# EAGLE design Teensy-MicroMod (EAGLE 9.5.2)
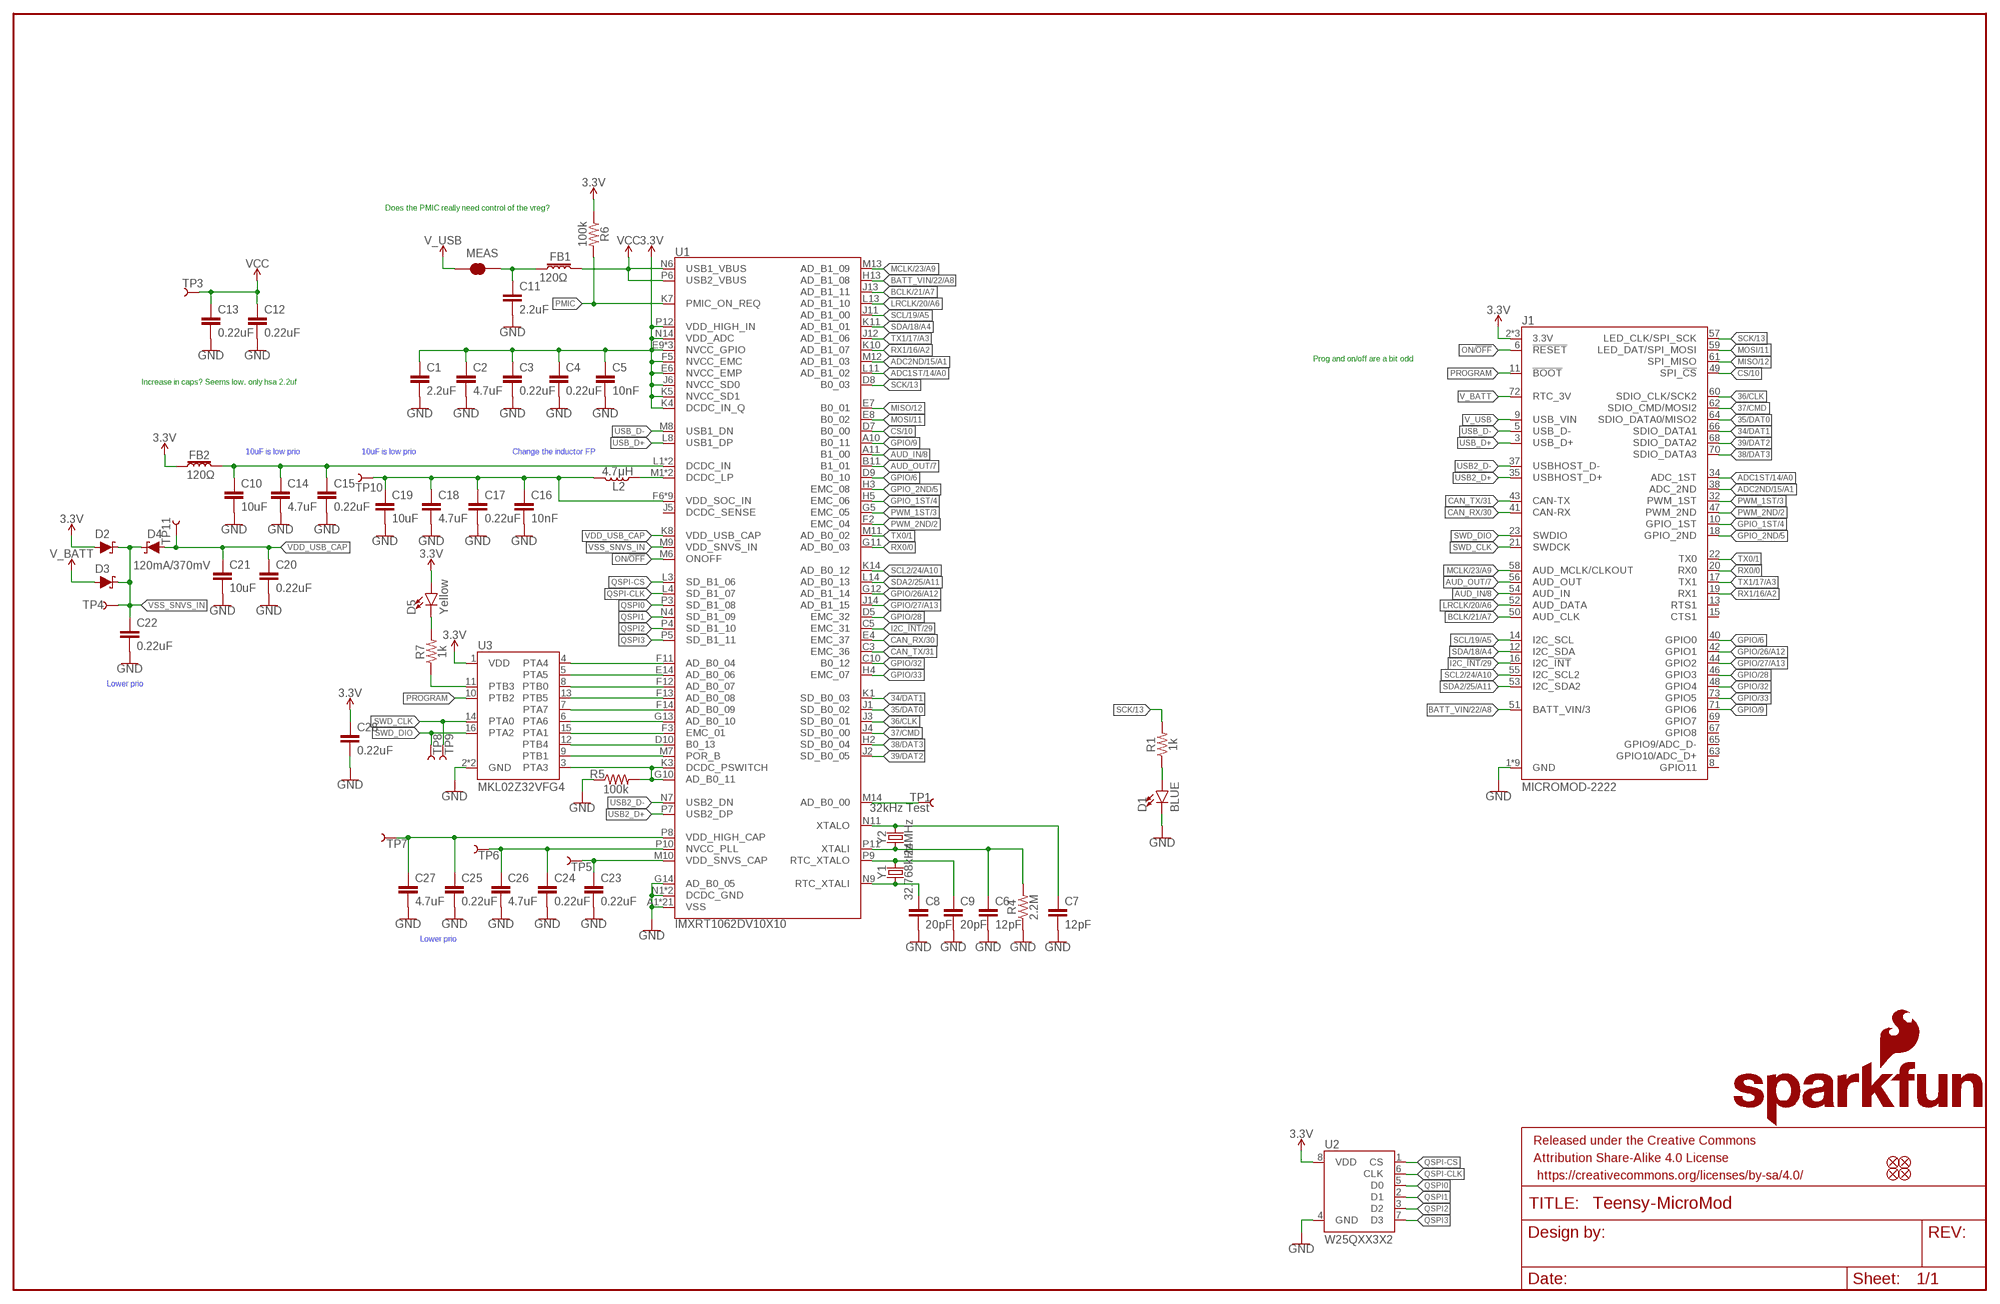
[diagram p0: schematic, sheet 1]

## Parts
C1  2.2uF  2.2UF-0402_TIGHT-10V-10%-X5R  [0402-TIGHT]
C2  4.7uF  4.7UF-0402_TIGHT-6.3V-20%-X5R  [0402-TIGHT]
C3  0.22uF  0.22UF-0402T-10V-10%  [0402-TIGHT]
C4  0.22uF  0.22UF-0402T-10V-10%  [0402-TIGHT]
C5  10nF  10NF-0402T-25V-10%  [0402-TIGHT]
C6  12pF  12PF-0402T-50V-5%  [0402-TIGHT]
C7  12pF  12PF-0402T-50V-5%  [0402-TIGHT]
C8  20pF  20PF-0402T-50V-5%  [0402-TIGHT]
C9  20pF  20PF-0402T-50V-5%  [0402-TIGHT]
C10  10uF  10UF-0402T-6.3V-20%  [0402-TIGHT]
C11  2.2uF  2.2UF-0402_TIGHT-10V-10%-X5R  [0402-TIGHT]
C12  0.22uF  0.22UF-0402T-10V-10%  [0402-TIGHT]
C13  0.22uF  0.22UF-0402T-10V-10%  [0402-TIGHT]
C14  4.7uF  4.7UF-0402_TIGHT-6.3V-20%-X5R  [0402-TIGHT]
C15  0.22uF  0.22UF-0402T-10V-10%  [0402-TIGHT]
C16  10nF  10NF-0402T-25V-10%  [0402-TIGHT]
C17  0.22uF  0.22UF-0402T-10V-10%  [0402-TIGHT]
C18  4.7uF  4.7UF-0402_TIGHT-6.3V-20%-X5R  [0402-TIGHT]
C19  10uF  10UF-0402T-6.3V-20%  [0402-TIGHT]
C20  0.22uF  0.22UF-0402T-10V-10%  [0402-TIGHT]
C21  10uF  10UF-0402T-6.3V-20%  [0402-TIGHT]
C22  0.22uF  0.22UF-0402T-10V-10%  [0402-TIGHT]
C23  0.22uF  0.22UF-0402T-10V-10%  [0402-TIGHT]
C24  0.22uF  0.22UF-0402T-10V-10%  [0402-TIGHT]
C25  0.22uF  0.22UF-0402T-10V-10%  [0402-TIGHT]
C26  4.7uF  4.7UF-0402_TIGHT-6.3V-20%-X5R  [0402-TIGHT]
C27  4.7uF  4.7UF-0402_TIGHT-6.3V-20%-X5R  [0402-TIGHT]
C28  0.22uF  0.22UF-0402T-10V-10%  [0402-TIGHT]
D1  BLUE  LED-BLUE0603  [LED-0603]
D2  120mA370mV  DIODE-SCHOTTKY-RB751S40  [SOD-523]
D3  120mA/370mV  DIODE-SCHOTTKY-RB751S40  [SOD-523]
D4  120mA/370mV  DIODE-SCHOTTKY-RB751S40  [SOD-523]
D5  Yellow  LED-YELLOW0603  [LED-0603]
FB1  120Ω  FERRITE_BEAD-120_OHM-0402  [0402]
FB2  120Ω  FERRITE_BEAD-120_OHM-0402  [0402]
FD1  FIDUCIALUFIDUCIAL  [FIDUCIAL-MICRO]
FD2  FIDUCIALUFIDUCIAL  [FIDUCIAL-MICRO]
FD3  FIDUCIALUFIDUCIAL  [FIDUCIAL-MICRO]
FD4  FIDUCIALUFIDUCIAL  [FIDUCIAL-MICRO]
FRAME1  FRAME-LEDGER  [CREATIVE_COMMONS]
J1  MICROMOD-2222  [M.2-CARD-E-22]
L2  4.7μH  4.7μH_SHIELDED_INDUCTOR  [1008(2520)]
LOGO1  SFE_LOGO_NAME_FLAME.1_INCH  [SFE_LOGO_NAME_FLAME_.1]
MEAS  JUMPER-SMT_2_NC_TRACE_SILK  [SMT-JUMPER_2_NC_TRACE_SILK]
R1  1k  1KOHM-0402T-1/16W-1%  [0402-TIGHT]
R4  2.2M  2.2MOHMS-0402T-1/10W-1%  [0402-TIGHT]
R5  100k  100KOHM-0402T-1/16W-1%  [0402-TIGHT]
R6  100k  100KOHM-0402T-1/16W-1%  [0402-TIGHT]
R7  1k  1KOHM-0402T-1/16W-1%  [0402-TIGHT]
TP1  32kHz Test  TEST-POINT2  [PAD.02X.02]
TP3  TEST-POINT2  [PAD.02X.02]
TP4  TEST-POINT2  [PAD.02X.02]
TP5  TEST-POINT2  [PAD.02X.02]
TP6  TEST-POINT2  [PAD.02X.02]
TP7  TEST-POINT2  [PAD.02X.02]
TP8  TEST-POINT2  [PAD.02X.02]
TP9  TEST-POINT2  [PAD.02X.02]
TP10  TEST-POINT2  [PAD.02X.02]
TP11  TEST-POINT2  [PAD.02X.02]
U1  IMXRT1062DV10X10  [IMXRT1062]
U2  W25QXX3X2  [USON-8]
U3  MKL02Z32VFG4  MKL02Z32VFG4QFN-16  [QFN-16]
Y1  32.768kHz  CRYSTAL-32.768KHZSMD-3.2X1.5  [CRYSTAL-SMD-3.2X1.5MM]
Y2  24MHz  CRYSTAL-24MHZ-SMD-2.0X1.6MM  [CRYSTAL-SMD-2.0X1.6MM]

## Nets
3.3V: C1.1 C2.1 C3.1 C4.1 C5.1 C28.1 D2.A D5.A FB2.1 J1.2(3.3V) J1.4(3.3V) J1.74(3.3V) R6.1 U1.E6(NVCC_EMP) U1.E9(NVCC_GPIO) U1.F5(NVCC_EMC) U1.F10(NVCC_GPIO) U1.J6(NVCC_SD0) U1.J10(NVCC_GPIO) U1.K4(DCDC_IN_Q) U1.K5(NVCC_SD1) U1.N14(VDD_ADC) U1.P12(VDD_HIGH_IN) U2.8(VDD) U3.1(VDD)
34/DAT1: J1.66(SDIO_DATA1) U1.K1(SD_B0_03)
35/DAT0: J1.64(SDIO_DATA0/MISO2) U1.J1(SD_B0_02)
36/CLK: J1.60(SDIO_CLK/SCK2) U1.J3(SD_B0_01)
37/CMD: J1.62(SDIO_CMD/MOSI2) U1.J4(SD_B0_00)
38/DAT3: J1.70(SDIO_DATA3) U1.H2(SD_B0_04)
39/DAT2: J1.68(SDIO_DATA2) U1.J2(SD_B0_05)
ADC1ST/14/A0: J1.34(ADC_1ST) U1.L11(AD_B1_02)
ADC2ND/15/A1: J1.38(ADC_2ND) U1.M12(AD_B1_03)
AUD_IN/8: J1.54(AUD_IN) U1.A11(B1_00)
AUD_OUT/7: J1.56(AUD_OUT) U1.B11(B1_01)
BATT_VIN/22/A8: J1.51(BATT_VIN/3) U1.H13(AD_B1_08)
BCLK/21/A7: J1.50(AUD_CLK) U1.J13(AD_B1_11)
BOOTMODE0: U1.F11(AD_B0_04) U3.4(PTA4)
CAN_RX/30: J1.41(CAN-RX) U1.E4(EMC_37)
CAN_TX/31: J1.43(CAN-TX) U1.C3(EMC_36)
CS/10: J1.49(SPI_!CS!) U1.D7(B0_00)
DEBUG_EN: U1.F3(EMC_01) U3.15(PTA1)
DEBUG_SWO: U1.D10(B0_13) U3.12(PTB4)
GND: C1.2 C2.2 C3.2 C4.2 C5.2 C6.2 C7.2 C8.2 C9.2 C10.2 C11.2 C12.2 C13.2 C14.2 C15.2 C16.2 C17.2 C18.2 C19.2 C20.2 C21.2 C22.2 C23.2 C24.2 C25.2 C26.2 C27.2 C28.2 D1.C J1.1(GND) J1.7(GND) J1.33(GND) J1.36(GND) J1.39(GND) J1.45(GND) J1.75(GND) J1.GND J1.GND-SM-B(GND) R4.1 R5.1 U1.A1(VSS) U1.A14(VSS) U1.B5(VSS) U1.B10(VSS) U1.E2(VSS) U1.E13(VSS) U1.G7(VSS) U1.G8(VSS) U1.G14(AD_B0_05) U1.H7(VSS) U1.H8(VSS) U1.J7(VSS) U1.J8(VSS) U1.K2(VSS) U1.K6(VSS) U1.K9(VSS) U1.K13(VSS) U1.L9(VSS) U1.N1(DCDC_GND) U1.N2(DCDC_GND) U1.N5(VSS) U1.N8(VSS) U1.P1(VSS) U1.P14(VSS) U2.4(GND) U3.2(GND) U3.17(GND)
GPIO/6: J1.40(GPIO0) U1.D9(B0_10)
GPIO/9: J1.71(GPIO6) U1.A10(B0_11)
GPIO/26/A12: J1.42(GPIO1) U1.G12(AD_B1_14)
GPIO/27/A13: J1.44(GPIO2) U1.J14(AD_B1_15)
GPIO/28: J1.46(GPIO3) U1.D5(EMC_32)
GPIO/32: J1.48(GPIO4) U1.C10(B0_12)
GPIO/33: J1.73(GPIO5) U1.H4(EMC_07)
GPIO_1ST/4: J1.10(GPIO_1ST) U1.H5(EMC_06)
GPIO_2ND/5: J1.18(GPIO_2ND) U1.H3(EMC_08)
I2C_!INT!/29: J1.16(I2C_!INT!) U1.C5(EMC_31)
JTAG_MOD: U1.F13(AD_B0_08) U3.13(PTB5)
JTAG_TCK: U1.F12(AD_B0_07) U3.8(PTB0)
JTAG_TDI: U1.F14(AD_B0_09) U3.7(PTA7)
JTAG_TDO: U1.G13(AD_B0_10) U3.6(PTA6)
JTAG_TMS: U1.E14(AD_B0_06) U3.5(PTA5)
JTAG_TRST: R5.2 U1.G10(AD_B0_11) U1.K3(DCDC_PSWITCH) U3.3(PTA3)
LRCLK/20/A6: J1.52(AUD_DATA) U1.L13(AD_B1_10)
MCLK/23/A9: J1.58(AUD_MCLK/CLKOUT) U1.M13(AD_B1_09)
MISO/12: J1.61(SPI_MISO) U1.E7(B0_01)
MOSI/11: J1.59(LED_DAT/SPI_MOSI) U1.E8(B0_02)
N$1: TP1.P$1 U1.M14(AD_B0_00)
N$2: D1.A R1.1
N$3: C10.1 C14.1 C15.1 FB2.2 U1.L1(DCDC_IN) U1.L2(DCDC_IN)
N$4: C7.1 U1.N11(XTALO) Y2.3
N$5: C6.1 R4.2 U1.P11(XTALI) Y2.1
N$9: L2.1 U1.M1(DCDC_LP) U1.M2(DCDC_LP)
N$10: C11.1 FB1.1 MEAS.2
N$12: R7.1 U3.11(PTB3)
N$13: D5.C R7.2
N$30: C23.1 TP5.P$1 U1.M10(VDD_SNVS_CAP)
N$31: C9.1 U1.P9(RTC_XTALO) Y1.P$2
N$32: C8.1 U1.N9(RTC_XTALI) Y1.P$1
N$33: C24.1 C26.1 TP6.P$1 U1.P10(NVCC_PLL)
N$34: C25.1 C27.1 TP7.P$1 U1.P8(VDD_HIGH_CAP)
ON/!OFF!: J1.6(!RESET!) U1.M6(ONOFF)
PMIC: R6.2 U1.K7(PMIC_ON_REQ)
PORB_RESET: U1.M7(POR_B) U3.9(PTB1)
PROGRAM: J1.11(!BOOT!) U3.10(PTB2)
PWM_1ST/3: J1.32(PWM_1ST) U1.G5(EMC_05)
PWM_2ND/2: J1.47(PWM_2ND) U1.F2(EMC_04)
QSPI0: U1.P3(SD_B1_08) U2.5(D0)
QSPI1: U1.N4(SD_B1_09) U2.2(D1)
QSPI2: U1.P4(SD_B1_10) U2.3(D2)
QSPI3: U1.P5(SD_B1_11) U2.7(D3)
QSPI-CLK: U1.L4(SD_B1_07) U2.6(CLK)
QSPI-CS: U1.L3(SD_B1_06) U2.1(CS)
RX0/0: J1.20(RX0) U1.G11(AD_B0_03)
RX1/16/A2: J1.19(RX1) U1.K10(AD_B1_07)
SCK/13: J1.57(LED_CLK/SPI_SCK) R1.2 U1.D8(B0_03)
SCL2/24/A10: J1.55(I2C_SCL2) U1.K14(AD_B0_12)
SCL/19/A5: J1.14(I2C_SCL) U1.J11(AD_B1_00)
SDA2/25/A11: J1.53(I2C_SDA2) U1.L14(AD_B0_13)
SDA/18/A4: J1.12(I2C_SDA) U1.K11(AD_B1_01)
SWD_CLK: J1.21(SWDCK) TP9.P$1 U3.14(PTA0)
SWD_DIO: J1.23(SWDIO) TP8.P$1 U3.16(PTA2)
TX0/1: J1.22(TX0) U1.M11(AD_B0_02)
TX1/17/A3: J1.17(TX1) U1.J12(AD_B1_06)
USB2_D+: J1.35(USBHOST_D+) U1.P7(USB2_DP)
USB2_D-: J1.37(USBHOST_D-) U1.N7(USB2_DN)
USB_D+: J1.3(USB_D+) U1.L8(USB1_DP)
USB_D-: J1.5(USB_D-) U1.M8(USB1_DN)
V_BATT: D3.A J1.72(RTC_3V)
V_USB: J1.9(USB_VIN) MEAS.1
VCC: C12.1 C13.1 FB1.2 TP3.P$1 U1.N6(USB1_VBUS) U1.P6(USB2_VBUS)
VDD_SOC_IN: C16.1 C17.1 C18.1 C19.1 L2.2 TP10.P$1 U1.F6(VDD_SOC_IN) U1.F7(VDD_SOC_IN) U1.F8(VDD_SOC_IN) U1.F9(VDD_SOC_IN) U1.G6(VDD_SOC_IN) U1.G9(VDD_SOC_IN) U1.H6(VDD_SOC_IN) U1.H9(VDD_SOC_IN) U1.J9(VDD_SOC_IN)
VDD_USB_CAP: C20.1 C21.1 D4.A TP11.P$1 U1.K8(VDD_USB_CAP)
VSS_SNVS_IN: C22.1 D2.C D3.C D4.C TP4.P$1 U1.M9(VDD_SNVS_IN)
Unconnected: J1.8(GPIO11) J1.13(RTS1) J1.15(CTS1) J1.63(GPIO10/ADC_D+) J1.65(GPIO9/ADC_D-) J1.67(GPIO8) J1.69(GPIO7) U1.J5(DCDC_SENSE)

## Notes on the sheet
- Does the PMIC really need control of the vreg?
- Prog and on/off are a bit odd
- Increase in caps? Seems low. only hsa 2.2uf
- 10uF is low prio | 10uF is low prio | Change the inductor FP
- Lower prio
- Lower prio

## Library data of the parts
C1 C11 = SparkFun-Capacitors:2.2UF: 2.2µF ceramic capacitors; PROD_ID: CAP-14232
C2 C14 C18 C26 C27 = SparkFun-Capacitors:4.7UF: 4.7µF ceramic capacitors; PROD_ID: CAP-14240
C3 C4 C12 C13 C15 C17 C20 C22-C25 C28 = SparkFun-Capacitors:0.22UF: 0.22µF ceramic capacitors; PROD_ID: CAP-14846
C5 C16 = SparkFun-Capacitors:10NF: 0.01uF/10nF/10,000pF ceramic capacitors; PROD_ID: CAP-14847
C6 C7 = SparkFun-Capacitors:12PF: 12pF ceramic capacitors; PROD_ID: CAP-14665
C8 C9 = SparkFun-Capacitors:20PF: 20pF ceramic capacitors; PROD_ID: CAP-14843
C10 C19 C21 = SparkFun-Capacitors:10UF: 10.0µF ceramic capacitors; PROD_ID: CAP-14848
D1 = SparkFun-LED:LED-BLUE: Blue SMD LED; PROD_ID: DIO-08575
D2-D4 = SparkFun-DiscreteSemi:DIODE-SCHOTTKY: Schottky diode; PROD_ID: DIO-11018; VALUE: 120mA/40V/370mV
D5 = SparkFun-LED:LED-YELLOW: Yellow SMD LED; PROD_ID: DIO-09003
FB1 FB2 = SparkFun-Coils:FERRITE_BEAD-120_OHM: Ferrite Bead (blocks, cores, rings, chokes, etc.); MFG_PART: BLM15HB121SN1D; PROD_ID: NDUC-14206
FD1-FD4 = SparkFun-Aesthetics:FIDUCIAL: Fiducial Alignment Points
FRAME1 = SparkFun-Aesthetics:FRAME-LEDGER: Schematic Frame - Ledger
J1 = Teensy:MICROMOD
L2 = SparkFun-Coils:4.7μH_SHIELDED_INDUCTOR: 4.7uH Inductor; PROD_ID: NDUC-14880
LOGO1 = SparkFun-Aesthetics:SFE_LOGO_NAME_FLAME: SparkFun Font Logo w/ Flame
MEAS = SparkFun-Jumpers:JUMPER-SMT_2_NC_TRACE: Normally closed trace jumper
R1 R7 = SparkFun-Resistors:1KOHM: 1kΩ resistor; PROD_ID: RES-14342
R4 = SparkFun-Resistors:2.2MOHMS: 2MΩ resistor; PROD_ID: RES-14844
R5 R6 = SparkFun-Resistors:100KOHM: 100kΩ resistor; PROD_ID: RES-13495
TP1 TP3-TP11 = SparkFun-Connectors:TEST-POINT: SparkFun Test Points
U1 = Teensy:IMXRT1062DV; PROD_ID: IC-14904
U2 = Teensy:W25QXX; PROD_ID: IC-14905
U3 = Teensy:MKL02Z32VFG4; PROD_ID: IC-14906
Y1 = SparkFun-Clocks:CRYSTAL-32.768KHZ: 32.768kHz Crystal; PROD_ID: XTAL-13062
Y2 = SparkFun-Clocks:CRYSTAL-24MHZ: 24MHz Crystal; PROD_ID: XTAL-14845

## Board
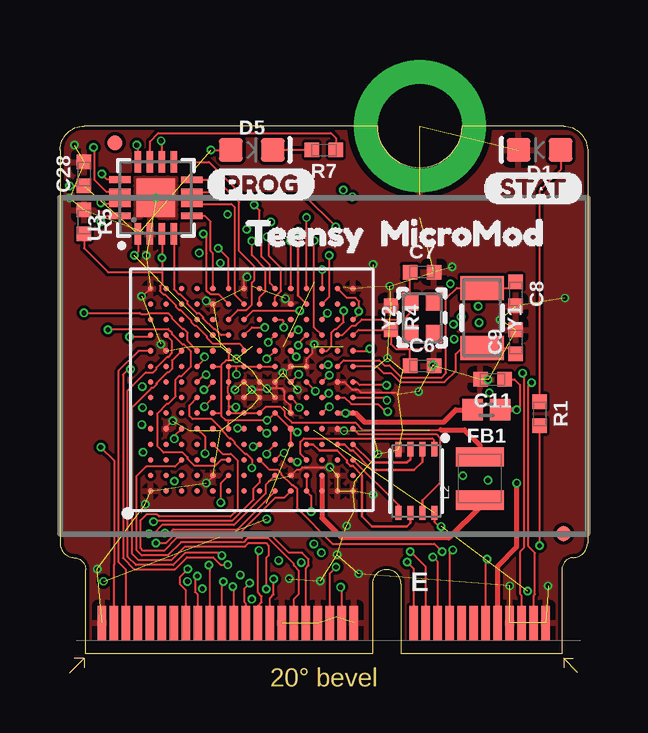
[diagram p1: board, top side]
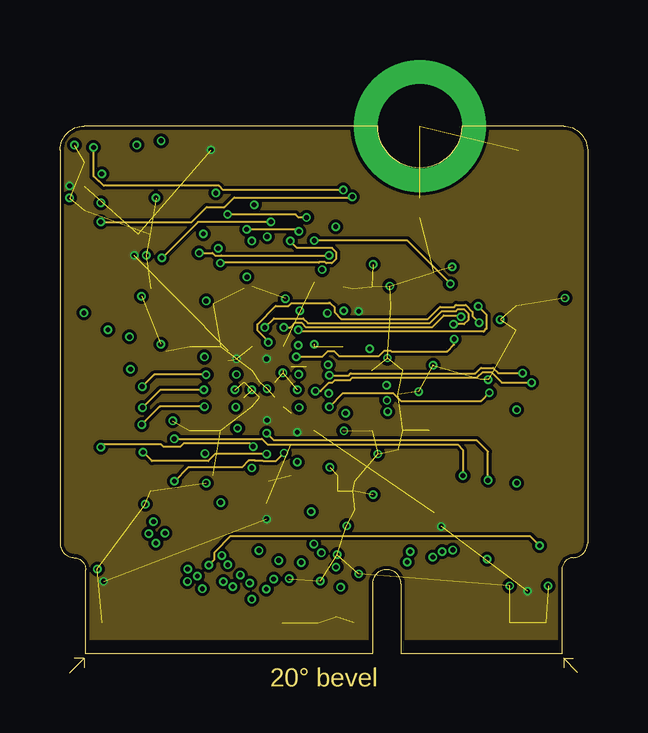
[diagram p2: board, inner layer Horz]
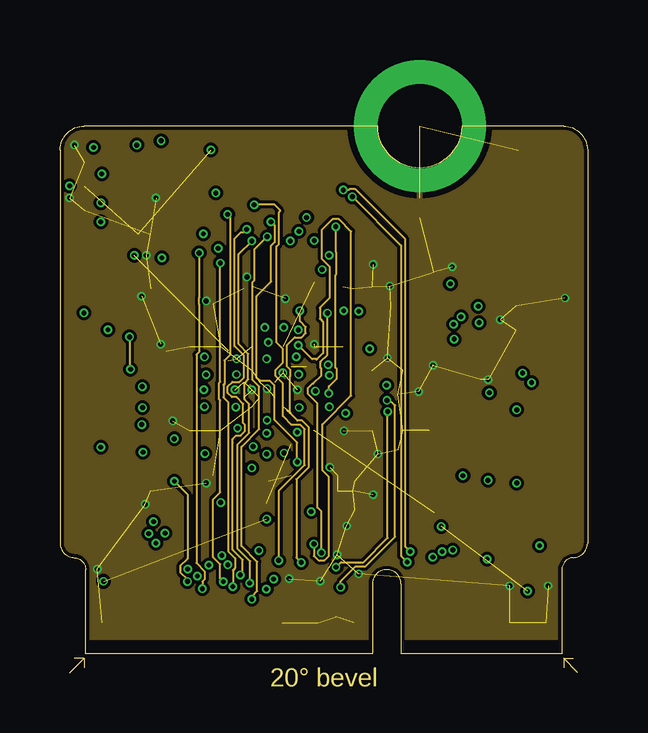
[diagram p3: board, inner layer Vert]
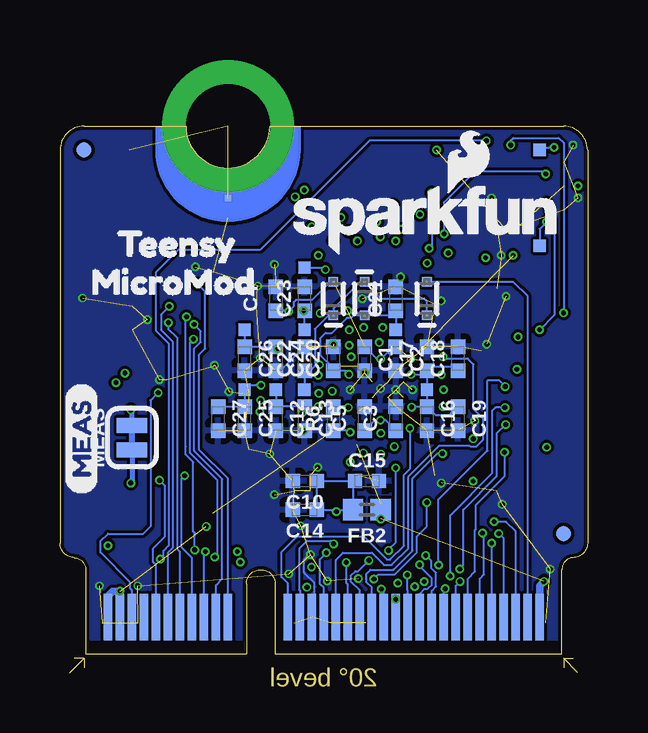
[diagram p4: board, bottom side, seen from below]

Size 22 x 22.8 mm. Coordinates in mm from the lower left corner, seen from the top.
Outline: 21.6,0 21,0.6
Outline: 21,0.6 21,0.2
Outline: 21,0.6 21.4,0.6
Outline: 0.4,0 1,0.6
Outline: 1,0.6 0.6,0.6
Outline: 1,0.6 1,0.2
Outline: 16.75,22.8 21,22.8 arc-87 22,21.8 22,5.4 arc-87 21.4,4.8 arc85 20.93,4.3 20.93,0.8 14.22,0.8 14.22,3.7 arc180 13.03,3.7 13.03,0.8 1.07,0.8 1.07,4.3 arc84 0.6,4.8 arc-87 0,5.4 0,21.8 arc-87 1,22.8 13.25,22.8
Outline: 16.75,22.8 arc-180 13.25,22.8
Outline: 16.75,22.8 arc-180 13.25,22.8
Copper layers (1+2*15+16): Top 0.035mm / dielectric 0.213359375mm / Horz 0.035mm / dielectric 1.0161mm / Vert 0.035mm / dielectric 0.213359375mm / Bottom 0.035mm
Design rules "SparkFun-4-layer-BGA-Extreme *": minimum track width 3.5mil, minimum drill 0.2mm, track to track 3.5mil, track to pad 3.5mil, pad to pad 3.5mil, via to via 3.5mil, smd to smd 0mil, copper to edge 4mil, drill to drill 4mil, minimum pad ring 3mil, minimum via ring 3mil, stop-mask expansion 4mil, vias tented up to drill 25mil, thermal gap 10mil

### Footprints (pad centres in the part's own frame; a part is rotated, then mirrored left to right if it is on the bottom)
0402-TIGHT = smd 0.6 x 0.6: 1 -0.5,0; 2 0.5,0
LED-0603 = smd 1 x 1: A -0.877,0; C 0.877,0
SOD-523 = smd 0.4 x 0.4: A -0.7,0; C 0.7,0
0402 = smd 0.85 x 0.9: 1 -0.58,0; 2 0.58,0
FIDUCIAL-MICRO = smd 0.635 x 0.635: 1 0,0
M.2-CARD-E-22 = smd 0.35 x 1.45: 1 9.25,1.275; 3 8.75,1.275; 5 8.25,1.275; 7 7.75,1.275; 9 7.25,1.275; 11 6.75,1.275; 13 6.25,1.275; 15 5.75,1.275; 17 5.25,1.275; 19 4.75,1.275; 21 4.25,1.275; 23 3.75,1.275; 33 1.25,1.275; 35 0.75,1.275; 37 0.25,1.275; 39 -0.25,1.275; 41 -0.75,1.275; 43 -1.25,1.275; 45 -1.75,1.275; 47 -2.25,1.275; 49 -2.75,1.275; 51 -3.25,1.275; 53 -3.75,1.275; 55 -4.25,1.275; 57 -4.75,1.275; 59 -5.25,1.275; 61 -5.75,1.275; 63 -6.25,1.275; 65 -6.75,1.275; 67 -7.25,1.275; 69 -7.75,1.275; 71 -8.25,1.275; 73 -8.75,1.275; 75 -9.25,1.275 | smd 0.35 x 1.95 bottom: 2 9,1.525; 4 8.5,1.525; 6 8,1.525; 8 7.5,1.525; 10 7,1.525; 12 6.5,1.525; 14 6,1.525; 16 5.5,1.525; 18 5,1.525; 20 4.5,1.525; 22 4,1.525; 32 1.5,1.525; 34 1,1.525; 36 0.5,1.525; 38 0,1.525; 40 -0.5,1.525; 42 -1,1.525; 44 -1.5,1.525; 46 -2,1.525; 48 -2.5,1.525; 50 -3,1.525; 52 -3.5,1.525; 54 -4,1.525; 56 -4.5,1.525; 58 -5,1.525; 60 -5.5,1.525; 62 -6,1.525; 64 -6.5,1.525; 66 -7,1.525; 68 -7.5,1.525; 70 -8,1.525; 72 -8.5,1.525; 74 -9,1.525 | drill 3.5 pad 5.5: GND 4,22 | smd 0.25 x 0.25 bottom: GND-SM-B 4,19
1008(2520) = smd 0.8 x 2: 1 -0.9,0; 2 0.9,0
SMT-JUMPER_2_NC_TRACE_SILK = smd 0.635 x 1.27: 1 -0.508,0; 2 0.508,0
PAD.02X.02 = smd 0.508 x 0.508: P$1 0,0
IMXRT1062 = smd 0.234 x 0.234: A1 -4.225,4.225; A2 -3.575,4.225; A3 -2.925,4.225; A4 -2.275,4.225; A5 -1.625,4.225; A6 -0.975,4.225; A7 -0.325,4.225; A8 0.325,4.225; A9 0.975,4.225; A10 1.625,4.225; A11 2.275,4.225; A12 2.925,4.225; A13 3.575,4.225; A14 4.225,4.225; B1 -4.225,3.575; B2 -3.575,3.575; B3 -2.925,3.575; B4 -2.275,3.575; B5 -1.625,3.575; B6 -0.975,3.575; B7 -0.325,3.575; B8 0.325,3.575; B9 0.975,3.575; B10 1.625,3.575; B11 2.275,3.575; B12 2.925,3.575; B13 3.575,3.575; B14 4.225,3.575; C1 -4.225,2.925; C2 -3.575,2.925; C3 -2.925,2.925; C4 -2.275,2.925; C5 -1.625,2.925; C6 -0.975,2.925; C7 -0.325,2.925; C8 0.325,2.925; C9 0.975,2.925; C10 1.625,2.925; C11 2.275,2.925; C12 2.925,2.925; C13 3.575,2.925; C14 4.225,2.925; D1 -4.225,2.275; D2 -3.575,2.275; D3 -2.925,2.275; D4 -2.275,2.275; D5 -1.625,2.275; D6 -0.975,2.275; D7 -0.325,2.275; D8 0.325,2.275; D9 0.975,2.275; D10 1.625,2.275; D11 2.275,2.275; D12 2.925,2.275; D13 3.575,2.275; D14 4.225,2.275; E1 -4.225,1.625; E2 -3.575,1.625; E3 -2.925,1.625; E4 -2.275,1.625; E5 -1.625,1.625; E6 -0.975,1.625; E7 -0.325,1.625; E8 0.325,1.625; E9 0.975,1.625; E10 1.625,1.625; E11 2.275,1.625; E12 2.925,1.625; E13 3.575,1.625; E14 4.225,1.625; F1 -4.225,0.975; F2 -3.575,0.975; F3 -2.925,0.975; F4 -2.275,0.975; F5 -1.625,0.975; F6 -0.975,0.975; F7 -0.325,0.975; F8 0.325,0.975; F9 0.975,0.975; F10 1.625,0.975; F11 2.275,0.975; F12 2.925,0.975; F13 3.575,0.975; F14 4.225,0.975; G1 -4.225,0.325; G2 -3.575,0.325; G3 -2.925,0.325; G4 -2.275,0.325; G5 -1.625,0.325; G6 -0.975,0.325; G7 -0.325,0.325; G8 0.325,0.325; G9 0.975,0.325; G10 1.625,0.325; G11 2.275,0.325; G12 2.925,0.325; G13 3.575,0.325; G14 4.225,0.325; H1 -4.225,-0.325; H2 -3.575,-0.325; H3 -2.925,-0.325; H4 -2.275,-0.325; H5 -1.625,-0.325; H6 -0.975,-0.325; H7 -0.325,-0.325; H8 0.325,-0.325; H9 0.975,-0.325; H10 1.625,-0.325; H11 2.275,-0.325; H12 2.925,-0.325; H13 3.575,-0.325; H14 4.225,-0.325; J1 -4.225,-0.975; J2 -3.575,-0.975; J3 -2.925,-0.975; J4 -2.275,-0.975; J5 -1.625,-0.975; J6 -0.975,-0.975; J7 -0.325,-0.975; J8 0.325,-0.975; J9 0.975,-0.975; J10 1.625,-0.975; J11 2.275,-0.975; J12 2.925,-0.975; J13 3.575,-0.975; J14 4.225,-0.975; K1 -4.225,-1.625; K2 -3.575,-1.625; K3 -2.925,-1.625; K4 -2.275,-1.625; K5 -1.625,-1.625; K6 -0.975,-1.625; K7 -0.325,-1.625; K8 0.325,-1.625; K9 0.975,-1.625; K10 1.625,-1.625; K11 2.275,-1.625; K12 2.925,-1.625; K13 3.575,-1.625; K14 4.225,-1.625; L1 -4.225,-2.275; L2 -3.575,-2.275; L3 -2.925,-2.275; L4 -2.275,-2.275; L5 -1.625,-2.275; L6 -0.975,-2.275; L7 -0.325,-2.275; L8 0.325,-2.275; L9 0.975,-2.275; L10 1.625,-2.275; L11 2.275,-2.275; L12 2.925,-2.275; L13 3.575,-2.275; L14 4.225,-2.275; M1 -4.225,-2.925; M2 -3.575,-2.925; M3 -2.925,-2.925; M4 -2.275,-2.925; M5 -1.625,-2.925; M6 -0.975,-2.925; M7 -0.325,-2.925; M8 0.325,-2.925; M9 0.975,-2.925; M10 1.625,-2.925; M11 2.275,-2.925; M12 2.925,-2.925; M13 3.575,-2.925; M14 4.225,-2.925; N1 -4.225,-3.575; N2 -3.575,-3.575; N3 -2.925,-3.575; N4 -2.275,-3.575; N5 -1.625,-3.575; N6 -0.975,-3.575; N7 -0.325,-3.575; N8 0.325,-3.575; N9 0.975,-3.575; N10 1.625,-3.575; N11 2.275,-3.575; N12 2.925,-3.575; N13 3.575,-3.575; N14 4.225,-3.575; P1 -4.225,-4.225; P2 -3.575,-4.225; P3 -2.925,-4.225; P4 -2.275,-4.225; P5 -1.625,-4.225; P6 -0.975,-4.225; P7 -0.325,-4.225; P8 0.325,-4.225; P9 0.975,-4.225; P10 1.625,-4.225; P11 2.275,-4.225; P12 2.925,-4.225; P13 3.575,-4.225; P14 4.225,-4.225
USON-8 = smd 0.6 x 0.25: 1 -1.325,0.75; 2 -1.325,0.25; 3 -1.325,-0.25; 4 -1.325,-0.75; 5 1.325,-0.75; 6 1.325,-0.25; 7 1.325,0.25; 8 1.325,0.75
QFN-16 = smd 0.9 x 0.29: 1 -1.5,0.75; 2 -1.5,0.25; 3 -1.5,-0.25; 4 -1.5,-0.75; 9 1.5,-0.75; 10 1.5,-0.25; 11 1.5,0.25; 12 1.5,0.75 | smd 0.29 x 0.9: 5 -0.75,-1.5; 6 -0.25,-1.5; 7 0.25,-1.5; 8 0.75,-1.5; 13 0.765,1.5; 14 0.25,1.5; 15 -0.25,1.5; 16 -0.75,1.5 | smd 1.6 x 1.6: 17 0,0
CRYSTAL-SMD-3.2X1.5MM = smd 1 x 1.8: P$1 -1.25,0; P$2 1.25,0
CRYSTAL-SMD-2.0X1.6MM = smd 0.75 x 0.7: 1 -0.675,-0.5; 2 0.675,-0.5; 3 0.675,0.5; 4 -0.675,0.5

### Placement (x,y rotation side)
C1  9.3,13.1 270 bottom
C2  8,13.1 270 bottom
C3  8,10.6 90 bottom
C4  13,15.6 90 bottom
C5  9.3,10.6 90 bottom
C6  15.1,12.8 0 top
C7  15.1,16.7 0 top
C8  19,15.8 270 top
C9  19,13.8 90 top
C10  11.8,8 180 bottom
C11  18.03,12.23 180 top
C12  13,10.6 270 bottom
C13  11.8,10.6 270 bottom
C14  11.8,6.8 180 bottom
C15  9.2,8 0 bottom
C16  6.7,10.6 270 bottom
C17  6.7,13.1 90 bottom
C18  5.4,13.1 90 bottom
C19  5.4,10.6 270 bottom
C20  10.6,13.1 90 bottom
C21  8,15.6 90 bottom
C22  11.8,13.1 90 bottom
C23  11.8,15.6 90 bottom
C24  13,13.1 270 bottom
C25  14.3,10.6 270 bottom
C26  14.3,13.1 270 bottom
C27  15.4,10.6 270 bottom
C28  1,20.8 90 top
D1  20,21.8 180 top
D2  10.6,15.6 270 bottom
D3  6.7,15.6 270 bottom
D4  9.3,15.6 90 bottom
D5  8,21.8 0 top
FB1  17.78,10.96 180 top
FB2  9.2,6.8 180 bottom
FD1  21,5.8 0 top
FD2  2.3,22.1 0 top
FD3  1,5.8 0 bottom
FD4  21,21.8 0 bottom
FRAME1  not placed on the board
J1  11,0.8 0 top
L2  17.5,8.1 90 top
LOGO1  6.7,18.9 0 bottom
MEAS  19,9.8 90 bottom
R1  20,10.8 270 top
R4  13.8,14.8 270 top
R5  1,18.8 270 top
R6  10.6,10.6 90 bottom
R7  11,21.8 180 top
TP1  11.8,16.9 270 bottom
TP3  13,11.8 90 bottom
TP4  11.81,11.8 0 bottom
TP5  11.8,14.3 0 bottom
TP6  14.3,14.3 0 bottom
TP7  14.3,11.8 0 bottom
TP8  2,17.8 0 bottom
TP9  2,21.8 0 bottom
TP10  6.7,11.8 270 bottom
TP11  8,14.3 270 bottom
U1  8,11.8 90 top
U2  14.86,7.99 270 top
U3  4,19.8 90 top
U$1  [TEENSY2]  20.5,17.9 0 bottom
U$2  [MICROMOD0]  12.45,18.33 0 top
U$3  [TEENSY2]  6.86,18.33 0 top
U$4  [PROG_32]  6.1,20.36 0 top
U$5  [MICROMOD0]  21.6,16.3 0 bottom
U$6  [STAT_32]  17.6,20.2 0 top
U$7  [MEAS_32]  21.1,7.4 90 bottom
Y1  17.6,14.8 270 top
Y2  15.1,14.8 90 top

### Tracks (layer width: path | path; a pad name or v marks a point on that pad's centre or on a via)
3.3V  (via drill 0.2)  (10 unrouted)
  Top 0.089: U1.K4 U1.K5 | 7,10.53 6.9,10.53 6.72,10.71 6.72,10.81 | 7,10.53 v8.63,10.53 8.68,10.53 U1.J6 U1.K5 | v7.37,13.09 | v8.62,13.09 U1.J10 | U1.N14 11.97,15.62 12.33,15.62 12.47,15.48 12.47,15.27 12.46,15.26 v12.46,15.07 12.46,14.96 U1.P12 | 6.72,12.76 6.72,12.83 6.92,13.03 7.02,13.03 | U1.E9 6.71,12.78 6.72,12.76 | 6.72,12.76 6.72,10.81 | U1.E6 6.71,10.83 6.72,10.81 | v7.37,13.09 7.31,13.03 7.02,13.03 | U1.F10 7.03,13.03 7.02,13.03 | v9.89,10.03 9.77,10.03 U1.K5 | U1.F5 7.03,10.51 7,10.53 | U2.8 15.61,6.29 15.8,6.1 v15.9,6.1 | C28.1 v0.4,20.3 | v6.3,21.8 D5.A | U3.1 3.25,17.55 v3.1,17.4
  Bottom 0.089: C5.1 8.87,10.53 v8.63,10.53 8.43,10.53 C3.1 | D2.A 10.73,16.3 11.49,15.54 12.16,15.54 12.24,15.46 12.24,15.29 v12.46,15.07 12.49,15.1 C4.1 | 8.62,7.05 FB2.1 v8.62,6.41 | C2.1 8.11,13.6 8.6,13.1 | 8.6,13.1 v8.62,13.09 | C1.1 8.8,13.1 8.6,13.1 | v8.62,6.41 | v9.89,10.03 9.96,10.1 R6.1
  Bottom 0.203: J1.4 v19.5,3.4 | J1.2 20,3.2
  Bottom 0.305: 20,3.2 19.8,3.4 v19.5,3.4 | v1.82,3.81 2,3.63 J1.74
  pour Horz (isolate 0.127): 0,1.4 0,22.8 22,22.8 22,1.4
34/DAT1  (via drill 0.2)
  Top 0.089: v4,5.4 4.4,5.4 4.8,5.8 7.47,5.8 8.97,7.3 9.35,7.3 U1.K1
  Bottom 0.089: J1.66 v4,5.4
35/DAT0  (via drill 0.2)
  Top 0.089: U1.J1 8.97,7.55 7.4,5.98 4.73,5.98 4.57,5.82 v4.38,5.82
  Bottom 0.089: v4.38,5.82 4.32,5.76 4.32,4.1 4.5,3.92 J1.64
36/CLK  (via drill 0.2)
  Top 0.089: U1.J3 9.27,9.17 v9.35,9.17
  Horz 0.089: v4.77,7.99 5.35,8.56 7.59,8.56 7.87,8.85 8.13,8.85 8.14,8.84 8.46,8.84 8.49,8.81 8.99,8.81 v9.35,9.17
  Vert 0.089: v4.77,7.99 5.32,7.44 5.32,4.75 5.02,4.45 5.02,4.19 5.32,3.89 v5.32,3.81
  Bottom 0.089: v5.32,3.81 5.5,3.63 J1.60
37/CMD  (via drill 0.2)
  Top 0.089: U1.J4 8.62,9.17 v8.62,9.12
  Horz 0.089: v8.62,9.12 6.47,9.12 6.18,8.83 3.83,8.83 v3.46,9.2
  Bottom 0.089: v3.46,9.2 3.46,8.19 4.67,6.99 4.67,5.97 4.69,5.95 4.69,4.22 5,3.91 J1.62
38/DAT3  (via drill 0.2)
  Top 0.089: U1.H2 8.32,7.93 8.07,7.68 8.07,7.22 7.19,6.33 3.93,6.33 v3.9,6.3
  Bottom 0.089: v3.9,6.3 3.4,6.3 3,5.9 J1.70
39/DAT2  (via drill 0.2)
  Top 0.089: U1.J2 8.57,7.83 8.57,7.47 7.26,6.16 4.26,6.16 3.9,5.8 v3.7,5.8
  Bottom 0.089: v3.7,5.8 3.5,5.6 J1.68
ADC1ST/14/A0  (via drill 0.2)
  Top 0.089: U1.L11 9.94,13.74 v9.94,13.66
  Vert 0.089: v10.59,5.37 10.59,4.87 10.77,4.69 11.03,4.69 11.21,4.87 11.21,8.17 10.95,8.44 10.95,10.36 12.14,11.55 12.14,18.4 11.63,18.91 11.37,18.91 10.91,18.45 10.91,17.27 11.24,16.94 11.24,15.62 10.84,15.22 10.84,14.77 10.97,14.63 10.97,13.33 10.72,13.08 | 10.72,13.08 10.69,13.04 | 10.72,13.08 10.51,13.08 v9.94,13.66
  Bottom 0.089: v10.59,5.37 10.59,5.39 10.7,5.5 11.7,5.5 12.01,5.19 12.01,3.44 12,3.43 J1.34
ADC2ND/15/A1  (via drill 0.2)
  Top 0.089: U1.M12 10.93,14.77 v11.15,14.99
  Vert 0.089: v10.9,5 10.9,6.73 10.74,6.89 10.74,11.23 10.35,11.62 10.35,11.87 10.53,12.06 10.55,12.06 10.9,12.4 10.9,12.69 10.87,12.71 10.87,12.97 11.15,13.25 v11.15,14.99
  Bottom 0.089: v10.9,5 11.17,4.73 11.17,3.7 11,3.53 J1.38
AUD_IN/8  (via drill 0.2)
  Top 0.089: v7,4.5 6.7,4.5 6.39,4.81 5.3,4.81 4.8,4.31 3.1,4.31 2.63,4.78 2.63,12.43 2.86,12.66 v2.94,12.66 | U1.A11 3.7,14 v2.9,14
  Vert 0.089: v2.9,14 2.9,12.7 v2.94,12.66
  Bottom 0.089: J1.54 7,3.29 6.8,3.49 6.68,3.49 6.5,3.67 6.5,3.93 7,4.43 v7,4.5
AUD_OUT/7  (via drill 0.2)
  Top 0.089: U1.B11 4.67,13.83 4.67,13.32 4.53,13.18 4.47,13.18 4.03,12.73 4.03,12.67 3.88,12.53 3.58,12.53 2.83,11.77 2.83,4.83 3.17,4.49 4.73,4.49 5.23,4.99 6.65,4.99 v6.75,4.89
  Bottom 0.089: v6.75,4.89 6.52,4.66 6.52,4.36 6.32,4.17 6.32,3.6 6.5,3.42 J1.56
BATT_VIN/22/A8  (via drill 0.2)
  Top 0.089: U1.H13 8.32,15.67 8.57,15.92 8.57,16.83 8,17.41 v8,18 | J1.51 7.75,2.88 7.69,2.94 7.69,3.52 v7.91,3.74
  Vert 0.089: v7.91,3.74 7.92,3.74 7.93,3.75 7.93,4.65 7.39,5.19 7.39,9.5 7.89,10 7.89,11.21 7.7,11.4 7.7,11.66 7.69,11.67 7.69,12.08 7.85,12.24 7.85,13.3 7.46,13.7 7.46,17.46 v8,18
BCLK/21/A7  (via drill 0.2)
  Top 0.089: U1.J13 8.97,15.67 9.22,15.92 9.22,16.88 8.7,17.4 8.7,18.12 v8.64,18.18
  Vert 0.089: v8,3.07 8,3.19 8.22,3.41 8.22,4.63 7.57,5.28 7.57,9.42 8.31,10.16 8.31,11.93 8.03,12.21 8.03,15.62 8.03,15.63 8.03,16.29 8.11,16.37 8.11,16.63 8.1,16.64 8.1,17.64 v8.64,18.18 8.62,18.18
  Bottom 0.089: J1.50 v8,3.07
BOOTMODE0
  Top 0.089: U1.F11 6.73,14.08 6.48,14.33 6.42,14.33 5.97,14.77 5.97,14.83 5.83,14.98 5.71,14.98 5.33,15.36 5.33,15.48 5.03,15.78 4.97,15.78 4.75,16 U3.4
CAN_RX/30
  Top 0.089: U1.E4 6.78,9.12 7.13,9.12 7.4,8.85 7.4,6.8 7.11,6.51 4.13,6.51 4.03,6.61 3.61,6.61 3.36,6.36 3.36,5.21 3.48,5.09 4.34,5.09 4.87,5.62 7.57,5.62 7.73,5.78 8.77,5.78 9.55,5 10.1,5 10.37,4.73 10.37,4.47 10.25,4.35 J1.41
CAN_TX/31
  Top 0.089: U1.C3 4.8,8.6 3.6,8.6 3.18,8.18 3.18,5.12 3.41,4.89 4.49,4.89 5.04,5.44 7.65,5.44 7.8,5.6 8.7,5.6 9.75,4.55 9.75,4.47 9.97,4.25 9.97,3.29 9.75,3.08 J1.43
CS/10  (via drill 0.2)
  Top 0.089: v8.3,5.1 8.25,5.05 8.25,3.35 8.41,3.19 8.41,2.94 8.25,2.78 J1.49 | v8,8.54 8,8.9 7.78,9.12 7.72,9.12 7.28,9.57 7.28,9.63 7.13,9.78 7.07,9.78 6.78,10.07 6.78,10.13 6.33,10.58 5.53,10.58 5.4,10.7 5.4,11.15 U1.D7
  Bottom 0.089: v8.3,5.1 8.3,5.14 8,5.44 v8,8.54
DEBUG_EN  (via drill 0.2)
  Top 0.089: U1.F3 6.73,8.88 6.48,8.62 5.62,8.62 5.33,8.92 5.33,8.98 5.12,9.18 4.32,9.18 4.06,9.44 4.06,10.82 4.47,11.23 4.53,11.23 4.83,11.52 4.83,12.23 4.97,12.38 5.08,12.38 5.46,12.76 5.46,13.39 5.18,13.68 5.12,13.68 4.67,14.12 4.67,14.18 4.51,14.34 2.04,14.34 v2,14.3 | U3.15 1.75,19.55 v1.7,19.6
  Bottom 0.089: v1.7,19.6 1.7,19.24 1.39,18.93 1.39,14.91 v2,14.3
DEBUG_SWO  (via drill 0.2)
  Top 0.089: U1.D10 5.33,13.83 5.33,14.18 5.18,14.33 5.12,14.33 4.67,14.77 4.67,14.83 4.53,14.98 3.67,14.98 3.66,14.96 3.37,14.96 3.33,15 v1,15 | U3.12 3.25,21.95 v3.2,22
  Bottom 0.089: v3.2,22 3.2,22.2 3.1,22.3 1.2,22.3 1,22.1 v1,15
GND  (via drill 0.2)  (87 unrouted)
  Top 0.089: U1.E2 6.38,8.19 v6.1,7.91 | U1.K6 9.62,11.12 9.38,11.37 9.38,11.75 9.27,11.85 9.02,11.85 | 9.02,11.85 v8.64,11.85 8.59,11.8 v8,11.8 | U1.J8 9.02,12.08 9.02,11.85 | U1.K9 9.35,12.5 v9.3,12.5 | U1.L9 10.28,13.07 10.53,13.32 10.53,13.62 v10.6,13.7 | U1.G14 7.67,16.38 v7.8,16.5 | U1.K13 v9.4,15.6 | U1.E13 6.22,15.38 v6.1,15.5 | U1.A14 3.45,15.7 v3.4,15.7 | U1.B10 4.2,13.65 v4.2,13.7 | U1.B5 4.42,10.23 v4.7,10.5 | U1.K2 9.88,8.47 10.02,8.47 10.11,8.56 v11.26,8.56 | U1.N5 11.66,10.09 v11.84,10.09 | U1.N8 11.87,12.12 12.18,11.81 12.42,11.81 12.55,11.68 14.02,11.68 14.1,11.6
  Bottom 0.089: C21.2 7.8,16.3 v7.8,16.5 | v11.56,4.92 11.62,4.92 11.82,4.73 11.82,4.17 11.39,3.74 11.39,2.44 J1.36 | C22.2 12.8,12.6 C24.2 | J1.GND-SM-B 15,18.97
  other vias: 3.56,7.02 3.6,17.4 4,19.8 0.4,19.8 0.6,22 13.06,7.42 11.96,6.12 10.86,3.82 9.56,3.92 12.46,4.12 1.56,4.32 20.36,3.62 21.06,15.62 18.36,14.72 16.36,16.92 15.56,12.82 17.86,12.22 13.66,13.12 18.76,3.62 13.26,9.12 7.3,11.8 9.9,11.8 14.96,11.72 13.06,17.02 13.76,16.12
  pour Bottom (isolate 0.127): 0,1.4 0,22.8 22,22.8 22,1.4
  pour Top (isolate 0.127): 0,1.4 0,22.8 22,22.8 22,1.4
  pour Vert (isolate 0.127): 0,1.4 0,22.8 22,22.8 22,1.4
GPIO/6  (via drill 0.2)
  Top 0.089: U1.D9 6.03,13.08 v6.03,13.17
  Bottom 0.089: v6.03,13.17 5.96,13.1 5,13.1 4.76,12.85 4.76,10.99 4.35,10.59 4.35,9.73 4.63,9.44 4.89,9.44 4.92,9.48 6.18,9.48 7.48,8.18 7.48,5.18 8.17,4.49 8.49,4.49 9,5 10.2,5 10.5,4.7 J1.40
GPIO/9
  Top 0.089: U1.A10 3.27,13.43 2.45,12.6 2.45,4.6 2.75,4.3 J1.71
GPIO/26/A12  (via drill 0.2)
  Top 0.089: U1.G12 8.05,15.1 v10,15.1
  Vert 0.089: 9.59,10.83 9.48,10.94 | v10.06,4.6 9.86,4.8 9.86,8.06 10.38,8.58 10.38,10.23 10.1,10.52 9.9,10.52 9.59,10.83 | v10,15.1 10,14.66 10.24,14.42 10.24,14.16 10.06,13.98 9.78,13.98 9.48,13.68 9.48,12.76 9.61,12.63 9.61,12.37 9.59,12.35 9.59,10.83
  Bottom 0.089: J1.42 10,3.68 10.04,3.72 10.04,4.58 v10.06,4.6
GPIO/27/A13  (via drill 0.2)
  Top 0.089: U1.J14 8.75,16.25 8.75,17 8.4,17.35 8.4,17.98 8.33,18.05 8.33,19.28 v8.1,19.51
  Vert 0.089: v9.12,4.68 9.12,7.57 10.2,8.66 10.2,10.16 10.02,10.34 9.66,10.34 9.3,10.7 9.3,12.06 8.99,12.37 8.99,12.63 9.3,12.94 9.3,13.5 9.02,13.78 9.02,17.77 9.13,17.88 9.13,19.19 9.2,19.26 8.95,19.51 v8.1,19.51
  Bottom 0.089: J1.44 9.5,3.43 9.87,3.79 9.87,4.05 9.68,4.23 9.57,4.23 v9.12,4.68
GPIO/28  (via drill 0.2)
  Top 0.089: U1.D5 6.05,9.85 v6.05,9.14
  Bottom 0.089: v6.05,9.14 6.26,9.14 7.3,8.1 7.3,5.09 8.1,4.29 9.06,4.29 9.22,4.13 9.22,3.77 9,3.55 J1.46
GPIO/32  (via drill 0.2)
  Top 0.089: U1.C10 4.67,13.03 4.67,12.67 4.53,12.53 4.47,12.53 4.03,12.08 4.03,12.02 3.88,11.88 3.82,11.88 3.01,11.06 3.01,4.96 3.27,4.69 4.64,4.69 5.22,5.27 7.72,5.27 7.86,5.41 8.59,5.41 8.7,5.3 8.7,4.89 8.6,4.79 v8.6,3.49
  Bottom 0.089: v8.6,3.49 8.5,3.39 J1.48
GPIO/33  (via drill 0.2)
  Top 0.089: U1.H4 8.23,9.43 v8.06,9.43 | v1.7,9.4 2.27,8.83 2.27,4.53 2.25,4.5 J1.73
  Horz 0.089: v1.7,9.4 1.81,9.51 4.23,9.51 4.31,9.43 5.03,9.43 5.17,9.58 7.91,9.58 v8.06,9.43
GPIO_1ST/4  (via drill 0.2)
  Top 0.089: U1.H5 8.44,10.18 v8.62,9.99
  Horz 0.089: v8.62,9.99 8.92,9.69 17.38,9.69 17.85,9.22 v17.85,8.02
  Bottom 0.089: v17.85,8.02 17.64,7.82 17.64,5.66 18.12,5.18 18.12,4.61 18,4.49 J1.10
GPIO_2ND/5  (via drill 0.2)
  Top 0.089: U1.H3 8.72,8.47 9.08,8.47 9.22,8.33 9.22,8.27 9.67,7.83 9.73,7.83 9.88,7.68 9.88,6.88 11.37,5.38 15.61,5.38 v15.94,5.05
  Bottom 0.089: v15.94,5.05 16,4.99 J1.18
I2C_!INT!/29  (via drill 0.2)
  Top 0.089: U1.C5 4.76,9.86 v4.76,9.75
  Horz 0.089: v4.76,9.75 8.42,9.75 8.66,9.51 16.59,9.51 16.8,9.3 v16.8,8.22
  Bottom 0.089: v16.8,8.22 16.93,8.09 16.93,5.23 16.5,4.8 J1.16
JTAG_MOD  (via drill 0.2)
  Top 0.089: U1.F13 6.62,15.78 6.27,15.78 6.12,15.92 6.12,17.49 6.11,17.5 6.11,18.17 v5.98,18.3 | U3.13 1.98,20.57 v1.74,20.8
  Bottom 0.089: v5.98,18.3 v5.99,18.29 | v5.99,18.29 6,18.28 | v1.74,20.8 1.84,20.9 4.7,20.9 5.99,19.61 v5.99,18.29
JTAG_TCK
  Top 0.089: U1.F12 7.42,15.12 7.78,15.12 8.01,15.36 8.01,16.27 8.11,16.37 8.11,16.95 7.48,17.58 7.48,19.62 6.55,20.55 U3.8
JTAG_TDI  (via drill 0.2)
  Top 0.089: U3.7 6.45,20.05 v6.5,20 | U1.F14 7.03,17.28 v6.6,17.7
  Bottom 0.089: v6.5,20 6.5,17.8 v6.6,17.7
JTAG_TDO
  Top 0.089: U3.6 7.15,19.55 7.3,19.4 7.3,15.75 U1.G13
JTAG_TMS
  Top 0.089: U3.5 6.05,19.05 6.29,18.81 6.29,17.57 6.38,17.49 U1.E14
JTAG_TRST  (via drill 0.2)
  Top 0.089: U3.3 v4.25,17.3 4.25,16.7 | 4.25,16.7 4.25,16.2 4.17,16.13 4.17,15.92 4.32,15.78 4.38,15.78 4.83,15.33 4.83,15.27 4.97,15.12 5.03,15.12 5.47,14.68 5.47,14.62 5.62,14.48 5.68,14.48 6.12,14.03 6.12,13.97 6.37,13.73 7.48,13.73 7.67,13.53 U1.G10 | R5.2 1,17.7 2,16.7 4.25,16.7 | U1.K3 9.8,8.88 v9.89,8.79
  Horz 0.089: v8.8,18.8 5.75,18.8 v4.25,17.3
  Vert 0.089: v9.89,8.79 9.89,9.59 8.95,10.54 8.95,11.72 8.95,11.98 8.76,12.16 8.34,12.16 8.21,12.29 8.21,15.7 8.2,15.7 8.81,16.31 8.81,17.81 8.95,17.95 8.95,18.65 v8.8,18.8
LRCLK/20/A6  (via drill 0.2)
  Top 0.089: v9.96,18.4 9.96,17.75 9.92,17.71
  Top 0.102: U1.L13 9.92,15.73 9.92,17.71
  Horz 0.089: v7.79,18.49 9.88,18.49 v9.96,18.4
  Vert 0.089: v7.79,18.49 7.67,18.37 7.55,18.37 7.28,18.1 7.28,13.62 7.67,13.23 7.67,12.31 7.49,12.12 7.19,12.12 6.99,11.93 6.99,11.67 7.17,11.49 7.36,11.49 7.64,11.21 7.64,10.41 7.72,10.33 7.72,10.07 7.54,9.89 7.35,9.89 7.2,9.74 7.2,9.6 | v7.52,4.08 7.62,4.17 7.62,4.71 7.2,5.13 7.2,9.6 | 7.2,9.6
  Bottom 0.089: v7.52,4.08 v7.52,4.07 7.52,3.46 7.5,3.44 J1.52
MCLK/23/A9  (via drill 0.2)
  Top 0.089: v11.22,17.41 v11.22,17.4 11.22,17.36 11.24,17.34 11.24,15.69 U1.M13
  Horz 0.089: v5.8,17.5 6.36,17.5 6.47,17.39 6.73,17.39 6.74,17.4 v11.22,17.4
  Vert 0.089: v5.94,3.5 5.94,3.8 6.04,3.9 6.04,4.23 5.69,4.57 5.69,13.27 5.8,13.38 5.8,15.36 5.79,15.37 5.79,15.63 5.8,15.64 v5.8,17.5
  Bottom 0.089: v5.94,3.5 6,3.44 J1.58
MISO/12  (via drill 0.2)
  Top 0.089: U1.E7 6.03,11.12 v6.03,11.1 | J1.61 5.25,3.44 5.01,3.68 5.01,4 v5.33,4.32
  Horz 0.089: v6.03,11.1 4.16,11.1 v3.41,10.35
  Bottom 0.089: v5.33,4.32 5.18,4.47 5.18,6.8 3.79,8.18 3.79,9.97 v3.41,10.35
MOSI/11  (via drill 0.2)
  Top 0.089: v5.73,4.03 5.63,3.93 5.63,3.37 5.75,3.25 J1.59 | U1.E8 6.05,11.8 v6,11.8
  Horz 0.089: v3.44,11.06 4.18,11.8 v6,11.8
  Bottom 0.089: v3.44,11.06 3.84,11.06 3.97,10.93 3.97,8.33 5.73,6.57 v5.73,4.03
N$1  (via drill 0.2)
  Top 0.089: v10.93,16.81 v10.93,16.8 U1.M14
  Bottom 0.089: TP1.P$1 11.02,16.9 v10.93,16.81
N$2
  Top 0.089: R1.1 20,20.1 20.9,21 20.9,21.78 D1.A
N$3  (via drill 0.2)
  Top 0.089: U1.L2 U1.L1 10.47,7.38 v10.47,6.72
  Bottom 0.089: C10.1 C15.1 9.78,7.92 FB2.2 10.39,6.8 v10.47,6.72 10.55,6.8 C14.1 C10.1
N$4
  Top 0.089: U1.N11 11.78,14.08 12.18,14.48 12.33,14.48 12.59,14.73 14.33,14.73 14.6,15 Y2.3 C7.1
N$5
  Top 0.089: U1.P11 12.45,14.3 R4.2 13.8,13.7 14,13.5 14.6,13.5 | 15.6,14.2 Y2.1 15.55,14.08 15.55,13.95 15.1,13.5 14.6,13.5 | C6.1 14.6,13.5
N$9
  Top 0.2: U1.M2 U1.M1 10.93,6.46 11.76,5.62 16.22,5.62 17.5,6.9 L2.1
N$10  (via drill 0.2)
  Top 0.089: FB1.1 18.39,10.99 18.41,10.96 | C11.1 18.95,12.23 19.18,12 19.18,11.09 v19.05,10.96
  Top 0.203: v19.05,10.96 18.41,10.96
  Bottom 0.203: MEAS.2 19,10.91 v19.05,10.96
N$12
  Top 0.089: U3.11 3.75,22.15 4.1,22.5 11.3,22.5 11.5,22.3 R7.1
N$13
  Top 0.089: R7.2 D5.C
N$30  (via drill 0.2)
  Top 0.089: U1.M10 11.13,13.43 11.32,13.62 11.32,14.18 11.47,14.33 11.53,14.33 11.82,14.62 v11.82,15.09 v11.83,15.09
  Bottom 0.089: C23.1 v11.83,15.09 11.8,15.06 TP5.P$1 | C23.1
N$31
  Top 0.089: C9.1 18.75,13.55 Y1.P$2 16.75,13.55 16.5,13.3 16.5,12.59 16.03,12.12 14.18,12.12 13.82,12.48 13.52,12.48 13.22,12.78 U1.P9
N$32
  Top 0.089: C8.1 18.75,16.05 Y1.P$1 16.55,16.05 16.1,15.6 16.1,12.5 15.9,12.3 14.25,12.3 13.74,12.81 13.53,12.81 13.32,13.03 11.82,13.03 U1.N9
N$33  (via drill 0.2)
  Top 0.089: U1.P10 12.84,13.43 v12.92,13.51
  Bottom 0.089: v12.92,13.51 C24.1 C26.1 TP6.P$1
N$34  (via drill 0.2)
  Top 0.089: U1.P8 12.36,12.12 12.49,11.99 v13.62,11.99
  Bottom 0.089: v13.62,11.99 14.11,11.99 TP7.P$1 C25.1 C27.1
ON/!OFF!  (via drill 0.2)
  Top 0.089: U1.M6 11.19,11.09 v11.23,11.09
  Horz 0.089: v11.23,11.09 11.81,11.66 13.89,11.66 14.21,11.34 17.57,11.34 v17.91,11.68
  Bottom 0.089: v17.91,11.68 18.22,11.36 18.22,6.1 18.52,5.8 20,5.8 20.31,5.49 20.31,5.01 19.07,3.77 19.07,3.5 19,3.43 J1.6
PMIC  (via drill 0.2)
  Top 0.089: U1.K7 9.97,11.13 v9.97,11.06
  Bottom 0.089: v9.97,11.06 10.01,11.1 R6.2
PORB_RESET  (via drill 0.2)
  Top 0.089: U3.9 6.21,21.3 7.61,19.9 10.2,19.9 v11.5,18.6 | U1.M7 11.04,11.48 v11.21,11.65
  Vert 0.089: v11.5,18.6 11.5,17.56 11.53,17.53 11.53,16.63 11.49,16.59 11.49,12.71 11.54,12.66 11.54,12.27 11.21,11.94 v11.21,11.65
PROGRAM  (via drill 0.2)
  Top 0.089: U3.10 4.25,22.15 v4.22,22.18 | J1.11 17.75,4.68 v17.81,4.74
  Bottom 0.089: v17.81,4.74 17.68,4.87 17.68,5.09 17.47,5.3 17.47,13.72 18.01,14.27 18.01,16.69 17.05,17.65 13.63,17.65 9.1,22.18 v4.22,22.18
PWM_1ST/3  (via drill 0.2)
  Top 0.089: U1.G5 7.43,10.18 v7.41,10.2
  Bottom 0.089: v7.41,10.2 v7.4,10.2 7.4,8.51 7.66,8.25 7.66,5.3 8.23,4.73 8.37,4.73 9.33,5.68 12.12,5.68 12.77,5.03 12.77,4 12.5,3.73 J1.32
PWM_2ND/2  (via drill 0.2)
  Top 0.089: U1.F2 6.7,7.9 v6.7,7.1 | v8.91,3.9 8.91,3.26 8.75,3.1 J1.47
  Bottom 0.089: v8.91,3.9 8.71,4.1 8.04,4.1 7.12,5.02 7.12,5.68 6.7,6.1 v6.7,7.1
QSPI0
  Top 0.102: U2.5 14.11,6.99 U1.P3
QSPI1
  Top 0.102: U1.N4 11.86,9.53 12.12,9.27 12.21,9.27 13.02,8.46 14.77,8.46 15.11,8.8 U2.2
QSPI2
  Top 0.102: U2.3 14.61,8.9 14.47,8.76 12.99,8.76 U1.P4
QSPI3
  Top 0.089: 15.87,7.94 15.87,9.77 15.69,9.95 12.45,9.95 U1.P5
  Top 0.102: U2.7 15.11,7.18 15.87,7.94
QSPI-CLK
  Top 0.102: U1.L4 10.56,9.53 10.82,9.27 11.54,9.27 11.97,8.85 11.97,8.77 12.12,8.62 12.21,8.62 12.6,8.23 12.6,6.51 13.01,6.11 14.47,6.11 14.61,6.25 U2.6
QSPI-CS
  Top 0.089: U2.1 15.61,9.69 15.52,9.78 10.17,9.78 10.03,9.63 10.03,9.12 U1.L3
RX0/0  (via drill 0.2)
  Top 0.089: U1.G11 8,14.4 v8.54,14.4
  Horz 0.089: v16.41,14.53 16.84,14.53 17.03,14.72 17.03,14.97 16.85,15.15 16.59,15.15 16.52,15.08 15.93,15.08 15.43,14.58 10.34,14.58 10.14,14.78 8.92,14.78 v8.54,14.4
  Bottom 0.089: v16.41,14.53 16.12,14.25 16.12,13.78 16.4,13.51 16.4,9.25 15.23,8.08 15.23,3.92 15.5,3.65 J1.20
RX1/16/A2  (via drill 0.2)
  Top 0.089: v15.55,4.82 15.75,4.62 J1.19 | U1.K10 9.85,13.2 v9.85,13.18
  Horz 0.089: v9.85,13.18 10.95,13.18 11.18,13.41 11.44,13.41 11.64,13.2 13.3,13.2 13.53,13.43 13.78,13.43 13.82,13.4 16.16,13.4 16.43,13.68 v16.43,13.91
  Bottom 0.089: v15.55,4.82 15.45,4.92 15.45,8.04 16.58,9.18 16.58,13.77 v16.43,13.91
SCK/13  (via drill 0.2)
  Top 0.089: v6.21,4.49 6.25,4.45 J1.57 | v20,5.3 R1.2 | U1.D8 6.03,12.43 v6.09,12.43
  Horz 0.089: v6.09,12.43 3.93,12.43 v3.43,11.93 | v6.21,4.49 6.44,4.72 6.44,5.02 7.12,5.7 19.6,5.7 v20,5.3
  Bottom 0.089: v6.21,4.49 6.21,7.23 4.17,9.27 4.17,12.18 3.68,12.18 v3.43,11.93
SCL2/24/A10  (via drill 0.2)
  Top 0.089: U1.K14 9.62,17.98 v9.6,18 | v6.81,3.8 6.75,3.74 J1.55
  Horz 0.089: v9.6,18 9.89,17.71 11.35,17.71 11.53,17.53 11.53,17.27 11.34,17.08 11.1,17.08 11.06,17.12 10.8,17.12 10.78,17.1 6.7,17.1 v6.68,17.08
  Vert 0.089: v6.81,3.8 6.68,3.92 6.68,4.52 6.39,4.81 6.39,7.23 6.68,7.52 6.68,11.36 6.63,11.41 6.63,12.08 6.68,12.12 v6.68,17.08
SCL/19/A5  (via drill 0.2)
  Top 0.089: U1.J11 8.69,13.79 v8.69,13.77
  Horz 0.089: v8.69,13.77 8.69,13.81 8.23,14.27 8.23,14.53 8.99,15.29 9.53,15.29 9.65,15.41 11.2,15.41 | 11.27,15.41 11.2,15.41 | v17.48,14.6 17.21,14.87 17.21,15.05 16.92,15.33 16.52,15.33 16.44,15.26 15.85,15.26 15.35,14.76 11.73,14.76 11.46,15.02 11.46,15.22 11.28,15.4 11.21,15.4 11.2,15.41
  Bottom 0.089: v17.48,14.6 17.48,14.34 17.11,13.97 17.11,5.16 17,5.05 J1.14
SDA2/25/A11  (via drill 0.2)
  Top 0.089: v7.21,3.59 7.25,3.55 J1.53 | U1.L14 v10.28,18.98
  Horz 0.089: v10.28,18.98 9.96,18.98 9.83,19.11 v6.99,19.11
  Vert 0.089: v6.99,19.11 7.1,19 7.1,13.26 6.86,13.02 6.86,12.05 6.81,12 6.81,11.49 7.02,11.28 7.02,5.06 7.31,4.77 7.31,4.37 7.21,4.27 v7.21,3.59
SDA/18/A4  (via drill 0.2)
  Top 0.089: v9.94,14.29 9.84,14.29 U1.K11
  Horz 0.089: v9.94,14.29 10,14.22 17.67,14.22 17.79,14.35 17.79,14.93 v17.45,15.28
  Bottom 0.089: v17.45,15.28 17.79,14.93 17.79,14.3 17.29,13.8 17.29,5.23 17.5,5.02 J1.12
SWD_CLK  (via drill 0.2)
  Top 0.089: U3.14 1.95,20.05 1.43,20.57 1.43,21.87 v1.4,21.9 | J1.21 15.25,4.41 v14.61,5.05
  Horz 0.089: v11.81,20.13 6.81,20.13 6.63,20.31 1.83,20.31 1.65,20.49 1.61,20.49 1.4,20.71 v1.4,21.9
  Vert 0.089: v14.61,5.05 14.4,5.25 14.4,18.08 12.32,20.16 12.06,20.16 12.03,20.13 v11.81,20.13
  Bottom 0.089: v1.4,21.9 1.9,21.9 TP9.P$1
SWD_DIO  (via drill 0.2)
  Top 0.089: U3.16 1.95,19.05 v1.7,18.8 | J1.23 14.75,4.34 v14.48,4.61
  Horz 0.089: v1.7,18.8 5.5,18.8 6.12,19.42 6.86,19.42 7.26,19.82 12.16,19.82 v12.19,19.85
  Vert 0.089: v14.48,4.61 14.22,4.86 14.22,17.82 v12.19,19.85
  Bottom 0.089: v1.7,18.8 2,18.5 TP8.P$1
TX0/1  (via drill 0.2)
  Top 0.089: U1.M11 10.6,14.4 v10.6,18.02
  Horz 0.089: v16.28,16.22 14.48,18.02 v10.6,18.02
  Bottom 0.089: v16.28,16.22 15.95,15.89 15.95,13.52 16.2,13.27 16.2,9.3 15,8.1 J1.22
TX1/17/A3  (via drill 0.2)
  Top 0.089: v16.38,5.12 16.25,4.98 J1.17 | U1.J12 9.27,14.73 9.33,14.66 v9.33,14.4
  Horz 0.089: v16.72,14.85 16.66,14.9 16,14.9 15.5,14.4 10.26,14.4 10.06,14.6 9.81,14.6 9.61,14.4 v9.33,14.4
  Bottom 0.089: v16.38,5.12 16.38,5.82 16.44,5.88 16.44,8.78 16.76,9.1 16.76,9.43 16.76,9.44 16.76,14.8 v16.72,14.85
USB2_D+  (via drill 0.2)
  Top 0.089: U1.P7 13.53,11.48 13.63,11.37 v13.63,11.35 | v11.7,3.57 11.7,3.46 11.75,3.42 J1.35
  Vert 0.089: v13.63,11.35 13.77,11.35 13.97,11.15 13.97,5.67 12.73,4.43 12.33,4.43 11.7,3.8 v11.7,3.57
USB2_D-  (via drill 0.2)
  Top 0.089: U1.N7 11.87,11.48 12.15,11.2 13.25,11.2 13.56,10.89 v13.66,10.89 | v11.51,4.4 11.25,4.14 J1.37
  Vert 0.089: v13.66,10.89 13.66,5.62 12.66,4.61 11.72,4.61 v11.51,4.4
USB_D+  (via drill 0.2)
  Top 0.089: U1.L8 v10.65,11.75 | v19.67,12.1 19.54,11.97 19.54,5.26 19.81,4.99 19.81,3.27 19.75,3.21 J1.3
  Horz 0.089: v10.65,11.75 10.87,11.75 11.21,12.09 11.36,12.09 11.47,12.2 12.1,12.2 12.2,12.3 17.4,12.3 17.63,12.53 17.98,12.53 18.42,12.1 v19.67,12.1
USB_D-  (via drill 0.2)
  Top 0.089: v19.29,12.49 19.36,12.43 19.36,5.22 19.19,5.05 19.19,3.27 19.25,3.21 J1.5 | U1.M8 11.2,12.4 v11.23,12.4
  Horz 0.089: v11.23,12.4 12.05,12.4 12.12,12.48 17.32,12.48 17.55,12.71 18.06,12.71 18.27,12.49 v19.29,12.49
V_BATT
  Bottom 0.089: D3.A 3.1,16.3 2.5,15.7 J1.72
V_USB  (via drill 0.2)
  Top 0.203: v19.05,7.91 19.05,5.25 18.25,4.45 J1.9
  Bottom 0.203: MEAS.1 19,7.96 v19.05,7.91
VCC  (via drill 0.2)
  Top 0.203: FB1.2 16.51,10.96 16,10.45 12.7,10.45 12.33,10.83 U1.P6 v11.91,10.83 U1.N6
  Bottom 0.089: v11.91,10.83 11.91,10.99 C13.1 C12.1 TP3.P$1
VDD_SOC_IN  (via drill 0.2)
  Top 0.089: 7.36,12.78 U1.G9 U1.H9 U1.J9 | 7.36,12.78 U1.F9 U1.F8 7.03,11.96 6.99,11.93 6.99,11.67 7.03,11.64 U1.F7 7.03,11.11 | 7.03,11.11 U1.F6 7.32,10.83 | 7.32,10.83 U1.G6 U1.H6 8.57,11.08 9.21,11.08 9.38,10.91 9.38,10.72 9.67,10.43 12.33,10.43 12.62,10.13 15.88,10.13 | v7.36,12.44 7.36,12.78 | 7.32,10.83 7.33,10.84 v7.33,11.08 7.05,11.08 7.03,11.11
  Top 0.2: 15.88,10.13 16.87,10.13 17.5,9.5 L2.2
  Bottom 0.089: C18.1 5.57,12.77 6.53,12.77 C17.1 | C17.1 TP10.P$1 C16.1 | v7.36,12.44 6.87,12.44 C17.1 | C16.1 6.72,11.08 v7.33,11.08 | C16.1 6.34,10.74 5.76,10.74 C19.1
VDD_USB_CAP  (via drill 0.2)
  Top 0.089: U1.K8 v9.94,12.44 v9.95,12.44
  Bottom 0.089: TP11.P$1 C21.1 8.2,14.9 D4.A 9.76,14.9 9.87,14.79 10.04,14.79 10.66,14.17 10.92,14.17 11.13,13.96 11.13,13.23 10.6,12.7 C20.1 10.1,12.6 v9.95,12.45 v9.95,12.44
VSS_SNVS_IN  (via drill 0.2)
  Top 0.089: v11.18,12.84 11.11,12.78 U1.M9
  Bottom 0.089: TP4.P$1 C22.1 | D3.C 6.72,14.92 6.72,15.51 6.82,15.61 8.61,15.61 D4.C 9.48,16.3 10.6,15.18 D2.C 10.8,14.9 11.37,14.33 11.37,12.8 | C22.1 | C22.1 11.56,12.84 | 11.3,12.84 v11.18,12.84 11.32,12.84 11.37,12.8 | C22.1 11.55,12.6 11.37,12.78 11.37,12.8

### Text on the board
Dimension: 20° bevel

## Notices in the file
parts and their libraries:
SparkFun-Aesthetics: Licensing: Creative Commons ShareAlike 4.0 International - https://creativecommons.org/licenses/by-sa/4.0
SparkFun-Aesthetics: Released under the Creative Commons Attribution Share-Alike 4.0 License
SparkFun-Aesthetics: https://creativecommons.org/licenses/by-sa/4.0
